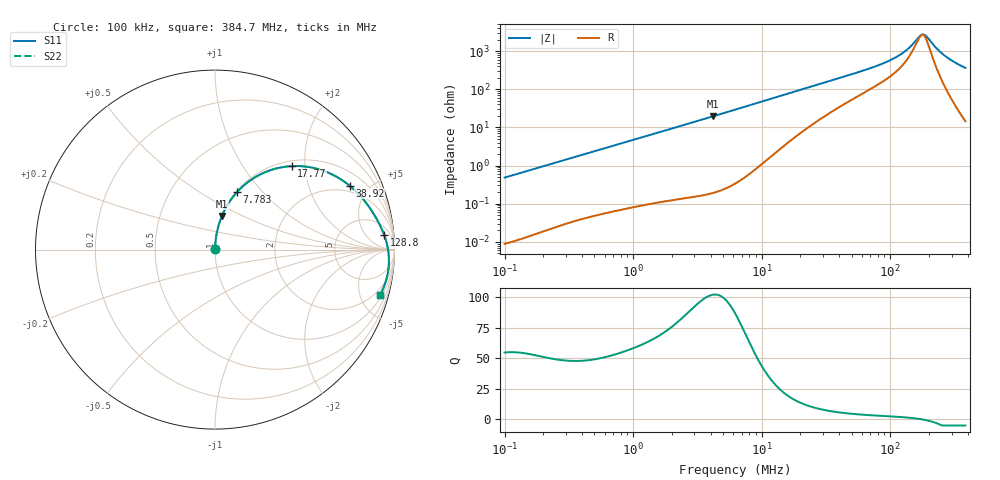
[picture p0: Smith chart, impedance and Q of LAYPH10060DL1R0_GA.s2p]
! LAYPH10060DL1R0_GA  S-PARAMETER MODEL  ( General Type )
! Model Generated by TAIYO YUDEN Corporation (http://www.ty-top.com)
! Version 3.0
! TAIYO YUDEN Control No. 180828NI43SB-FBB
! Copyright(c) 2017 TAIYO YUDEN CO.,LTD. All Rights Reserved.
! Product Description (link to TY-COMPAS)
! https://ds.yuden.co.jp/TYCOMPAS/or/detail?pn=LAYPH10060DL1R0NGA&u=M
! Products Name : Inductors
! Characteristics :
!  Inductance : 1.0 uH , SRF(min) : -Hz , DC Resistance(max) : 0.006 Ohm
!  Rated Current : Saturation :9.7 A , Temp Rise : 6 A (25 degC)
!  Case Size : 10.1 x 10.0 / 0.398 x 0.394 [mm/inch] , Thickness : 6 / 0.236 [mm/inch]
!  (Conditions: Temperature = 25 degC , DC Bias Current/Voltage = 0A / 0V)
! External Node Assignments :
!  1  o---GGG---o  2
! GND o---------o GND
! Frequency Range : 0.1MHz  -  384.651195MHz  [ 402 STEP ]
# MHz S RI R 50
! Freq[MHz].  S11 Real  S11 Imag  S21 Real  S21 Imag  S12 Real  S12 Imag  S22 Real  S22 Imag
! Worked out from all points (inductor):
!   401 points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, 100 kHz to 384.7 MHz, reference 50 ohm
!   read as one part in series: L = 767 nH near 104.2 kHz
!   highest Q = 102 at 4.19 MHz (marker M1), where L = 742 nH
!   self-resonance near 176.8 MHz
!   S11 on the Smith chart (normalised r, x): 100 kHz: 1.00, +0.01; 7.783 MHz: 1.01, +0.73; 17.77 MHz: 1.10, +1.71; 38.92 MHz: 1.64, +3.76; 128.8 MHz: 11, +17; 384.7 MHz: 1.29, -7.26
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0.1  0.000111 0.00482  0.9999 -0.00482  0.9999 -0.00482  0.000111 0.00482
0.398565  0.000752 0.0189  0.9992 -0.0189  0.9992 -0.0189  0.000752 0.0189
1.588538  0.00653 0.0736  0.9935 -0.0736  0.9935 -0.0736  0.00653 0.0736
4.190278  0.0385 0.1875  0.9615 -0.1875  0.9615 -0.1875  0.0385 0.1875
6.331348  0.0836 0.271  0.9164 -0.271  0.9164 -0.271  0.0836 0.271
7.782567  0.1221 0.3199  0.8779 -0.3199  0.8779 -0.3199  0.1221 0.3199
11.51897  0.2377 0.4113  0.7623 -0.4113  0.7623 -0.4113  0.2377 0.4113
17.76763  0.4278 0.4651  0.5722 -0.4651  0.5722 -0.4651  0.4278 0.4651
24.71908  0.5827 0.4461  0.4173 -0.4461  0.4173 -0.4461  0.5827 0.4461
38.92342  0.7497 0.3565  0.2503 -0.3565  0.2503 -0.3565  0.7497 0.3565
67.95212  0.8679 0.2242  0.1321 -0.2242  0.1321 -0.2242  0.8679 0.2242
98.5215  0.9161 0.1417  0.0839 -0.1417  0.0839 -0.1417  0.9161 0.1417
128.8385  0.9429 0.0806  0.0571 -0.0806  0.0571 -0.0806  0.9429 0.0806
145.8215  0.9528 0.0505  0.0472 -0.0505  0.0472 -0.0505  0.9528 0.0505
168.4847  0.9619 0.0131  0.0381 -0.0131  0.0381 -0.0131  0.9619 0.0131
175.5843  0.964 0.00189  0.036 -0.00189  0.036 -0.00189  0.964 0.00189
182.9831  0.9657 -0.00951  0.0343 0.00951  0.0343 0.00951  0.9657 -0.00951
194.67  0.9677 -0.0271  0.0323 0.0271  0.0323 0.0271  0.9677 -0.0271
229.6151  0.9689 -0.0765  0.0311 0.0765  0.0311 0.0765  0.9689 -0.0765
265.3011  0.9643 -0.1226  0.0357 0.1226  0.0357 0.1226  0.9643 -0.1226
319.4501  0.9489 -0.1854  0.0511 0.1854  0.0511 0.1854  0.9489 -0.1854
384.6512  0.921 -0.2506  0.079 0.2506  0.079 0.2506  0.921 -0.2506
